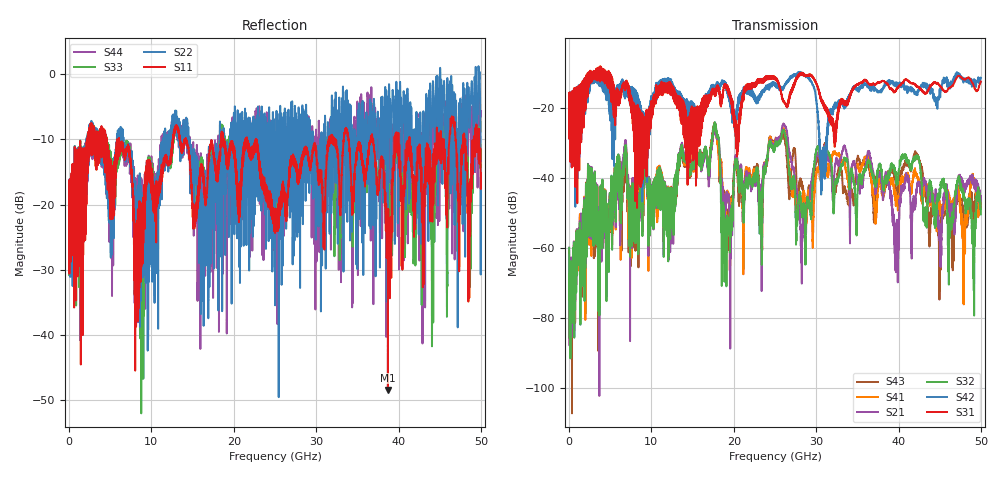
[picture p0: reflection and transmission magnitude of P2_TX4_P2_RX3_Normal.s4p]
!Keysight Technologies,N5225B,MY57041031,A.13.20.10
!Date: Friday, May 31, 2019 11:31:01
!Correction: S11(Full 4 Port(1,2,3,4))
!S12(Full 4 Port(1,2,3,4))
!S13(Full 4 Port(1,2,3,4))
!S14(Full 4 Port(1,2,3,4))
!S21(Full 4 Port(1,2,3,4))
!S22(Full 4 Port(1,2,3,4))
!S23(Full 4 Port(1,2,3,4))
!S24(Full 4 Port(1,2,3,4))
!S31(Full 4 Port(1,2,3,4))
!S32(Full 4 Port(1,2,3,4))
!S33(Full 4 Port(1,2,3,4))
!S34(Full 4 Port(1,2,3,4))
!S41(Full 4 Port(1,2,3,4))
!S42(Full 4 Port(1,2,3,4))
!S43(Full 4 Port(1,2,3,4))
!S44(Full 4 Port(1,2,3,4))
!S4P File: Measurements: <S11,S12,S13,S14>,
!<S21,S22,S23,S24>,
!<S31,S32,S33,S34>,
!<S41,S42,S43,S44>:
# Hz S  dB  R 50.0
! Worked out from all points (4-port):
!   5000 points, 10 MHz to 50 GHz, reference 50 ohm
!   strongest paths, dB at 10 MHz, 12.51 GHz, 25.01 GHz, 37.51 GHz, 50 GHz:
!     S31: -19.3, -14.3, -11.3, -12.8, -12.5
!     S42: -19.4, -14.3, -13.2, -15.6, -11.4
!     S32: -60.0, -46.7, -31.0, -38.4, -50.5
!     S21: -60.1, -47.0, -30.0, -39.2, -46.5
!     S41: -60.8, -46.0, -29.6, -43.8, -47.0
!     S43: -74.3, -45.8, -29.4, -38.0, -45.9
!   lowest |S11| = -48.5 dB at 38.71 GHz (marker M1), VSWR 1.01, Z = 49.6 - j0.129 ohm
!   |S11| at or under -10 dB: 6.073 GHz to 12.61 GHz (6.542 GHz wide, 70 % of centre); 14.21 GHz to 18.43 GHz (4.227 GHz wide, 25.9 % of centre); 22.71 GHz to 31.52 GHz (8.807 GHz wide, 32.5 % of centre)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
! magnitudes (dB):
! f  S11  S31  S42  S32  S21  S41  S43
! 10 MHz  -19.0  -19.3  -19.4  -60.0  -60.1  -60.8  -74.3
! 17.66 GHz  -13.4  -15.7  -14.3  -24.5  -25.7  -24.9  -24.2
! 19.03 GHz  -11.5  -13.7  -14.3  -56.1  -45.1  -45.7  -51.9
! 26.03 GHz  -18.9  -18.3  -14.0  -26.2  -24.5  -25.9  -27.5
! 28.41 GHz  -12.3  -10.2  -10.4  -47.7  -52.3  -44.7  -43.1
! 38.71 GHz  -48.5  -13.5  -12.6  -40.8  -41.6  -39.7  -38.1
! 50 GHz  -15.2  -12.5  -11.4  -50.5  -46.5  -47.0  -45.9
